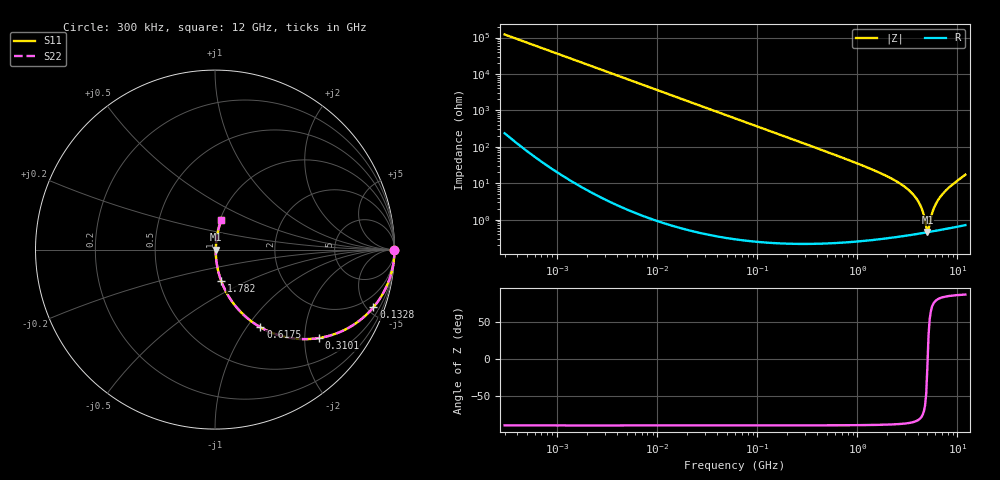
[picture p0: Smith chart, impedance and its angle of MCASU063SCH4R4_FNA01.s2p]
! MCASU063SCH4R4_FNA01  S-PARAMETER MODEL  ( General Type )
! Model Generated by TAIYO YUDEN Corporation (http://www.ty-top.com)
! Version 1.0
! TAIYO YUDEN Control No. 130801
! Copyright(c) 2013 TAIYO YUDEN CO.,LTD. All Rights Reserved.
! Product Description (link to TY-COMPAS)
! https://ds.yuden.co.jp/TYCOMPAS/or/detail?pn=MCASU063SCH4R4CFNA01&u=M
! Products Name : Multilayer Ceramic Capacitors
! Characteristics :
!  Capacitance : 4.4 pF , Rated Voltage : 50V , TCC : CH / C0H
!  Case Size : 0.6 x 0.3 / 0.024 x 0.012 [mm/inch] , Thickness : 0.3 / 0.012 [mm/inch]
!  (Conditions: Temperature = 25 degC , DC Bias Current/Voltage = 0A / 0V)
! External Node Assignments :
!  1  o---| |---o  2
! GND o---------o GND
! Frequency Range : 0.3MHz  -  12000MHz  [ 401 STEP ]
# MHz S RI R 50
! Freq[MHz].  S11 Real  S11 Imag  S21 Real  S21 Imag  S12 Real  S12 Imag  S22 Real  S22 Imag
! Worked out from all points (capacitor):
!   401 points, 300 kHz to 12 GHz, reference 50 ohm
!   read as one part in series: C = 4.37 pF near 316.3 kHz
!   lowest |Z| = 459 mohm at 5.006 GHz (marker M1)
!   series resonance near 5.037 GHz, so ESL is about 230 pH
!   S11 on the Smith chart (normalised r, x): 300 kHz: open; 132.8 MHz: 1.00, -5.48; 310.1 MHz: 1.00, -2.34; 617.5 MHz: 1.00, -1.16; 1.782 GHz: 1.01, -0.36; 12 GHz: 1.01, +0.34
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0.3  1 -0.000823  2.28e-06 0.000823  2.28e-06 0.000823  1 -0.000823
1.769972  1 -0.00486  2.54e-05 0.00486  2.54e-05 0.00486  1 -0.00486
10.44266  0.9992 -0.0286  0.000828 0.0286  0.000828 0.0286  0.9992 -0.0286
60  0.9735 -0.1603  0.0265 0.1603  0.0265 0.1603  0.9735 -0.1603
132.8329  0.8823 -0.3218  0.1177 0.3218  0.1177 0.3218  0.8823 -0.3218
310.0777  0.578 -0.493  0.422 0.493  0.422 0.493  0.578 -0.493
353.9943  0.5119 -0.4988  0.4881 0.4988  0.4881 0.4988  0.5119 -0.4988
617.4538  0.2534 -0.433  0.7466 0.433  0.7466 0.433  0.2534 -0.433
994.7115  0.112 -0.3118  0.888 0.3118  0.888 0.3118  0.112 -0.3118
1781.601  0.0337 -0.1724  0.9663 0.1724  0.9663 0.1724  0.0337 -0.1724
2088.533  0.0234 -0.1406  0.9766 0.1406  0.9766 0.1406  0.0234 -0.1406
2947.191  0.0101 -0.0802  0.9899 0.0802  0.9899 0.0802  0.0101 -0.0802
3740.715  0.00582 -0.0432  0.9942 0.0432  0.9942 0.0432  0.00582 -0.0432
4270.516  0.00474 -0.0238  0.9953 0.0238  0.9953 0.0238  0.00474 -0.0238
4502.883  0.00454 -0.0161  0.9955 0.0161  0.9955 0.0161  0.00454 -0.0161
4875.354  0.00446 -0.00466  0.9955 0.00466  0.9955 0.00466  0.00446 -0.00466
5006.236  0.0045 -0.000835  0.9955 0.000835  0.9955 0.000835  0.0045 -0.000835
5278.635  0.00465 0.0064  0.9954 -0.0064  0.9954 -0.0064  0.00465 0.0064
5868.704  0.0053 0.0212  0.9947 -0.0212  0.9947 -0.0212  0.0053 0.0212
6699.894  0.00685 0.0407  0.9932 -0.0407  0.9932 -0.0407  0.00685 0.0407
8503.825  0.0125 0.081  0.9875 -0.081  0.9875 -0.081  0.0125 0.081
12000  0.0353 0.165  0.9647 -0.165  0.9647 -0.165  0.0353 0.165
